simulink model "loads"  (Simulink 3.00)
settings: Solver=ode45  SolverMode=SingleTasking  StartTime=0.0  StopTime=10.0  RelTol=1e-3  AbsTol=1e-6

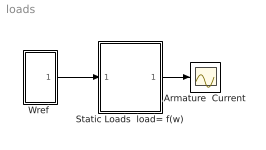
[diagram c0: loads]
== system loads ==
  Armature  Current : Scope
  Static Loads  load= f(w) : Subsystem  mask(Load Torques){w=1, Tn=1, c=Piston Compresors}
      mask prompts: w "Rated Speed [rad/sec]:"; Tn "Rated Torque [N*m]:"; c "Load Type:"
      mask help: This block generates at its output a Load torque which is a function of the rotational speed. The block icon displays the load characteristic in use. The left edge of the icon represents the load from 0 to 100% of ratred load, and the lower edge represents the speed from 0 to 100% rated speed.
      mask init:
      | switch c
      | case 1
      | x=[0  1];
      | y=[1 1];
      | case 2
      | x=[0 1 1.5 2 3 4 5 6 10];
      | y=[1.22 .98 .91 .92 .95 .97 .98 1 1];
      | case 3
      | x=[0 1 2 3 4 5 6 7 8 9 10];
      | y=[1 .87 .84 .85 .88 .9 .92 .94 .96 .98 1];
      | case 4
      | x=[0 1 2 3 4 5 6 7 8 9 10];
      | y=[1.3 1.1 .98 .95 .94 .945 .95 .96 .97 .98 1];
      | case 5
      | x=[0 1 2 3 4 5 6 7 8 9 10];
      | y=[1.3 1.1 .98 .95 .94 .945 .95 .96 .97 .98 1];
      | case 6
      | x=[0 1 2 3 4 5 6 7 8 9 10];
      | y=[.5 .36 .34 .36 .44 .5 .6 .7 .8 .9 1];
      | case 7
      | x=[0 .5 .50001 1 2 3 4 5 6 7 8 9 10];
      | y=[0 0 .08 .05 .04 .1 .17 .24 .36 .47 .62 .8 1];
      | case 8
      | x=[0 .5 .50001 1 2 3 4 5 6 7 8 9 10];
      | y=[0 0 .08 .05 .04 .1 .17 .24 .36 .47 .62 .8 1];
      | end
  "Wref " : Subsystem  mask(Slope Generator){ti=1, Tr=1, K=1}
      mask prompts: ti "Initial Time [sec]:"; Tr "Rise Time [sec]:"; K "Final Value:"
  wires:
  "Wref "/1(slope) -> Static Loads  load= f(w)/1(In)
  Static Loads  load= f(w)/1(Out1) -> Armature  Current/1

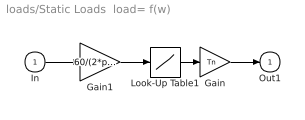
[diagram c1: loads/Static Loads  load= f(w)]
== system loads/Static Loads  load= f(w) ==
  In : Inport  Port=1  PortWidth=-1  SampleTime=-1  DataType=auto
  Gain : Gain  Gain=Tn  SaturateOnIntegerOverflow=on
  Gain1 : Gain  Gain=60/(2*pi*w)  SaturateOnIntegerOverflow=on
  Look-Up Table1 : Lookup  InputValues=x  OutputValues=y
  Out1 : Outport  Port=1  InitialOutput=0
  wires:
  Look-Up Table1/1 -> Gain/1
  Gain/1 -> Out1/1
  In/1 -> Gain1/1
  Gain1/1 -> Look-Up Table1/1

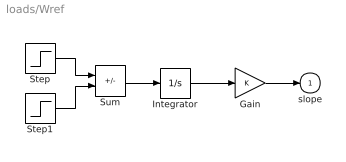
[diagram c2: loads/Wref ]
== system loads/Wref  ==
  Gain : Gain  Gain=K  SaturateOnIntegerOverflow=on
  Integrator : Integrator  ExternalReset=none  InitialConditionSource=internal  InitialCondition=0  LimitOutput=off  UpperSaturationLimit=inf  LowerSaturationLimit=-inf  ShowSaturationPort=off  ShowStatePort=off  AbsoluteTolerance=auto
  Step : Step  Time=ti  Before=0  After=1/Tr  SampleTime=0
  Step1 : Step  Time=ti+Tr  Before=0  After=1/Tr  SampleTime=0
  Sum : Sum  Inputs=+-  SaturateOnIntegerOverflow=on
  slope : Outport  Port=1  InitialOutput=0
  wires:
  Integrator/1 -> Gain/1
  Gain/1 -> slope/1
  Sum/1 -> Integrator/1
  Step/1 -> Sum/1
  Step1/1 -> Sum/2
